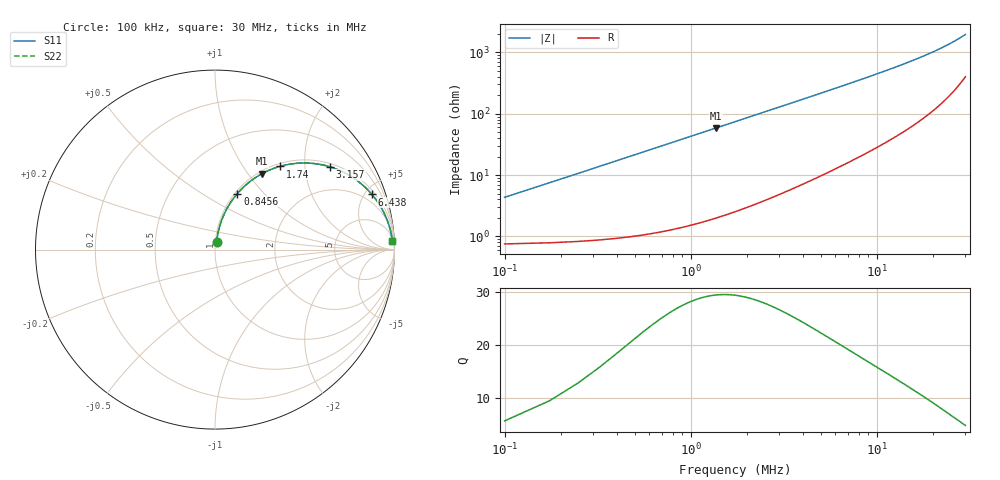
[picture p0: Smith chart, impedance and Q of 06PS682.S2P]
! Coilcraft 0603PS-682 Power Chip Inductor
! 19 February 2003
# MHZ S MA R 50
!Freq  MagS11  AngS11  MagS21  AngS21  MagS12  AngS12  MagS22  AngS22
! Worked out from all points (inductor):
!   403 points, 100 kHz to 30 MHz, reference 50 ohm
!   read as one part in series: L = 6.8 uH near 249.1 kHz
!   highest Q = 29.4 at 1.368 MHz (marker M1), where L = 6.8 uH
!   S11 on the Smith chart (normalised r, x): 100 kHz: 1.02, +0.09; 845.6 kHz: 1.03, +0.72; 1.74 MHz: 1.05, +1.49; 3.157 MHz: 1.10, +2.71; 6.438 MHz: 1.28, +5.58; 30 MHz: 9, +38
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0.1  0.04302 77.6  0.9916 -2.4  0.9916 -2.4  0.04302 77.6
0.17456  0.0742 79.7  0.9895 -4.2  0.9895 -4.2  0.0742 79.7
0.24912  0.1053 79.5  0.9863 -6.0  0.9863 -6.0  0.1053 79.5
0.32368  0.1361 78.6  0.9821 -7.8  0.9821 -7.8  0.1361 78.6
0.39824  0.1665 77.3  0.977 -9.6  0.977 -9.6  0.1665 77.3
0.4728  0.1964 75.9  0.971 -11.3  0.971 -11.3  0.1964 75.9
0.62192  0.2544 72.9  0.9565 -14.7  0.9565 -14.7  0.2544 72.9
0.8456  0.336 68.3  0.9295 -19.6  0.9295 -19.6  0.336 68.3
1.06928  0.4104 63.8  0.8977 -24.2  0.8977 -24.2  0.4104 63.8
1.36752  0.4975 58.2  0.8507 -29.8  0.8507 -29.8  0.4975 58.2
1.74032  0.5877 52.1  0.7894 -36.0  0.7894 -36.0  0.5877 52.1
2.41136  0.7059 43.1  0.6837 -44.9  0.6837 -44.9  0.7059 43.1
3.15696  0.7901 35.7  0.5836 -52.1  0.5836 -52.1  0.7901 35.7
4.05168  0.8522 29.3  0.4893 -58.4  0.4893 -58.4  0.8522 29.3
5.09552  0.8951 24.0  0.4072 -63.4  0.4072 -63.4  0.8951 24.0
6.4376  0.9269 19.3  0.3317 -67.8  0.3317 -67.8  0.9269 19.3
8.00336  0.9478 15.7  0.2704 -71.1  0.2704 -71.1  0.9478 15.7
10.09104  0.9632 12.4  0.2146 -74.0  0.2146 -74.0  0.9632 12.4
15.08656  0.9789 7.9  0.1384 -77.3  0.1384 -77.3  0.9789 7.9
20.08208  0.9848 5.5  0.09677 -78.2  0.09677 -78.2  0.9848 5.5
25.0776  0.9874 4.0  0.0697 -77.6  0.0697 -77.6  0.9874 4.0
30  0.9885 2.8  0.05046 -75.4  0.05046 -75.4  0.9885 2.8
